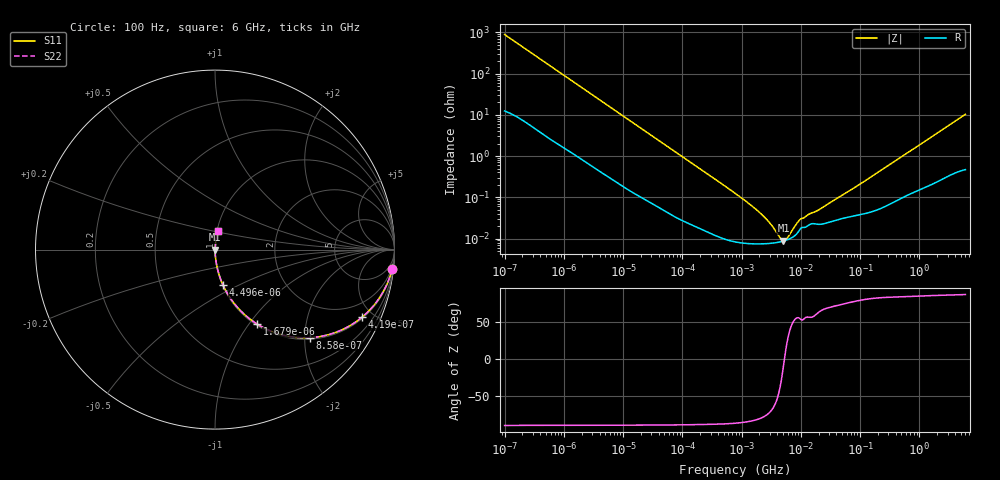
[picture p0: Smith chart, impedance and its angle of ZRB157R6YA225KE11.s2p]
!Murata Part Number: ZRB157R6YA225KE11
!These Parameters are Measured in Series Mode Connection
!Data Generated on Jun 10, 2025
!  o--ll--o
!Port1  Port2
!  o------o
!Operation Temp=25[degC], DC Bias Voltage=0[V]
!Freq. Start=100[Hz] Stop=6[GHz] 401[Steps]
# Hz S RI R 50
!Freq.(Hz) S11(Real) S11(Imag) S21(Real) S21(Imag) S12(Real) S12(Imag) S22(Real) S22(Imag)
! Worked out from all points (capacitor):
!   401 points, 100 Hz to 6 GHz, reference 50 ohm
!   read as one part in series: C = 1.78 uF near 109 Hz
!   lowest |Z| = 8.82 mohm at 5.079 MHz (marker M1)
!   series resonance near 5.285 MHz, so ESL is about 510 pH
!   S11 on the Smith chart (normalised r, x): 100 Hz: 1, -18; 419 Hz: 1.07, -4.32; 858 Hz: 1.04, -2.13; 1.679 kHz: 1.02, -1.10; 4.496 kHz: 1.01, -0.41; 6 GHz: 1.01, +0.21
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100  0.986 -0.1105  0.014 0.1105  0.014 0.1105  0.986 -0.1105
224  0.9383 -0.2325  0.0617 0.2325  0.0617 0.2325  0.9383 -0.2325
419  0.8198 -0.3762  0.1802 0.3762  0.1802 0.3762  0.8198 -0.3762
858  0.5305 -0.4906  0.4695 0.4906  0.4695 0.4906  0.5305 -0.4906
1174  0.3806 -0.4768  0.6194 0.4768  0.6194 0.4768  0.3806 -0.4768
1679  0.2348 -0.4151  0.7652 0.4151  0.7652 0.4151  0.2348 -0.4151
2008  0.1784 -0.374  0.8216 0.374  0.8216 0.374  0.1784 -0.374
4496  0.0444 -0.1969  0.9556 0.1969  0.9556 0.1969  0.0444 -0.1969
11514  0.00819 -0.0809  0.9918 0.0809  0.9918 0.0809  0.00819 -0.0809
40335  0.00112 -0.0236  0.9989 0.0236  0.9989 0.0236  0.00112 -0.0236
774597  8.46e-05 -0.00126  0.9999 0.00126  0.9999 0.00126  8.46e-05 -0.00126
2169299  7.44e-05 -0.000382  0.9999 0.000382  0.9999 0.000382  7.44e-05 -0.000382
3103719  7.66e-05 -0.00021  0.9999 0.00021  0.9999 0.00021  7.66e-05 -0.00021
4246196  8.17e-05 -8.33e-05  0.9999 8.33e-05  0.9999 8.33e-05  8.17e-05 -8.33e-05
5079039  8.69e-05 -1.5e-05  0.9999 1.5e-05  0.9999 1.5e-05  8.69e-05 -1.5e-05
6075234  9.48e-05 5.31e-05  0.9999 -5.31e-05  0.9999 -5.31e-05  9.48e-05 5.31e-05
9506416  0.000161 0.000233  0.9998 -0.000233  0.9998 -0.000233  0.000161 0.000233
1.555665e7  0.000229 0.000353  0.9998 -0.000353  0.9998 -0.000353  0.000229 0.000353
7.129496e7  0.000344 0.0015  0.9997 -0.0015  0.9997 -0.0015  0.000344 0.0015
3.124326e8  0.000709 0.00613  0.9993 -0.00613  0.9993 -0.00613  0.000709 0.00613
1.791126e9  0.00322 0.0321  0.9968 -0.0321  0.9968 -0.0321  0.00322 0.0321
6e9  0.0151 0.1011  0.9849 -0.1011  0.9849 -0.1011  0.0151 0.1011
